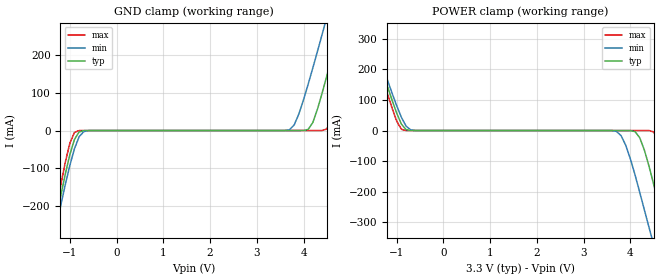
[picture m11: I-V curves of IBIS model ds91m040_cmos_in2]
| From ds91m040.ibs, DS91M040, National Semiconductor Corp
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|   Model  ds91m040_cmos_in2
[Model]   ds91m040_cmos_in2
Model_type Input
Vinh=2.0
Vinl=0.8
|   Typ   Min   Max
C_comp   1.809pF   1.767p   1.852pF
[Model Spec]
S_overshoot_high   3.3   3.0   3.6
S_overshoot_low   0.0   0.0   0.0
[Temperature Range]   25   85   -40
[Voltage Range]   3.3   3.0   3.6
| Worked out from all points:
|   GND clamp passes 1 mA (typ) near -0.72 V on its own axis
|   POWER clamp passes 1 mA (typ) near -0.73 V on its own axis
[GND Clamp]
-3.3V     -1.43A     -1.381A    -1.496A
-1.4V     -300.2mA   -317mA     -282.4mA
-1.3V     -238.5mA   -259.5mA   -215.4mA
-1V       -64.23mA   -92.67mA   -34.04mA
-800mV    -3.54mA    -16.35mA   -129.2uA
3.7V      1.298uA    2.184mA    432nA
4.1V      2.977mA    122.6mA    2.251uA
4.4V      99.81mA    255.1mA    77.6uA
4.5V      145.1mA    300.6mA    4.128mA
4.8V      287.3mA    438.8mA    121.9mA
5.1V      433.4mA    578.6mA    273.4mA
6.5V      1.128A     1.24A      1.009A
[POWER Clamp]
-3.3V     1.178A     1.145A     1.062A
-1.6V     335.7mA    346.4mA    325mA
-900mV    21.35mA    43.52mA    4.128mA
-600mV    5.153uA    139.5uA    2.729uA
3.7V      -3.097uA   -2.688mA   -5.254uA
3.9V      -12.03uA   -48.06mA   -5.255uA
4.2V      -23.47mA   -201.9mA   -5.275uA
4.4V      -117.2mA   -317mA     -129.2uA
4.5V      -176.8mA   -374.4mA   -4.736mA
4.8V      -361.6mA   -545.5mA   -148.6mA
5.1V      -544.3mA   -715mA     -349mA
6.5V      -1.372A    -1.381A    -1.247A
